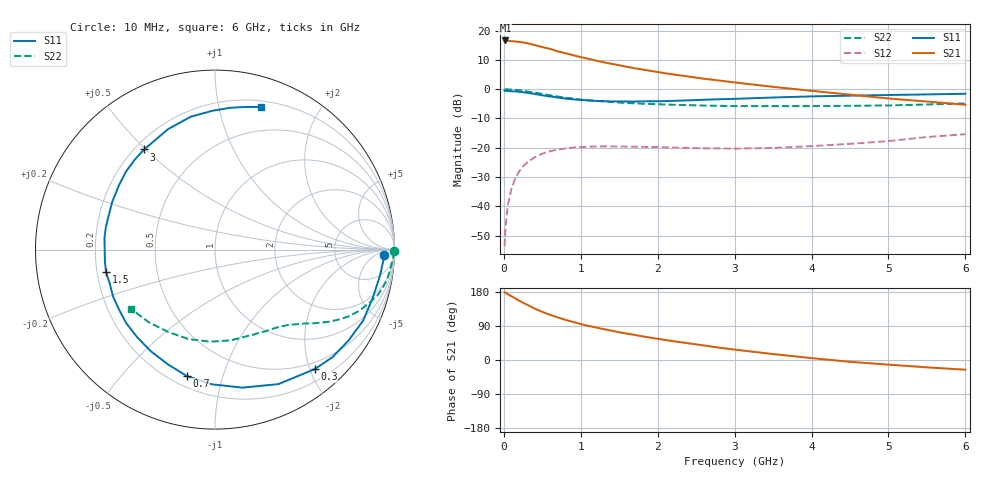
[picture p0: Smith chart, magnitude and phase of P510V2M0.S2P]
! SIEMENS Small Signal Semiconductors
! BFP183
! Si NPN RF Bipolar Junction Transistor in SOT143
! VCE = 10 V  IC = 2 mA
! Common Emitter S-Parameters:  March  1996
# GHz  S  MA  R  50
!  f  S11  S21  S12  S22
! GHz  MAG  ANG  MAG  ANG  MAG  ANG  MAG  ANG
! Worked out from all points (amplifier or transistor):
!   36 points, 10 MHz to 6 GHz, reference 50 ohm
!   highest |S21| = 16.6 dB at 20 MHz (marker M1)
!   |S21| within 3 dB of that: start of sweep to 614.7 MHz
!   unconditionally stable (mu >= 1): 2.182 GHz to 5.881 GHz
!   at 250 MHz: K = 0.11, MSG = 21.2 dB, |S12| = -26.4 dB
!   at 1.4 GHz: K = 0.65, MSG = 14.1 dB, |S12| = -19.5 dB
!   at 6 GHz: K = 0.98, MSG = 5.0 dB, |S12| = -15.4 dB
!   S11 on the Smith chart (normalised r, x): 10 MHz: 26, -12; 300 MHz: 0.39, -2.08; 700 MHz: 0.26, -0.77; 1.5 GHz: 0.24, -0.10; 3 GHz: 0.24, +0.49; 6 GHz: 0.26, +1.34
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0.01  0.9394 -1.7  6.732 178.9  0.0021 81.8  0.9972 -0.6
0.02  0.9401 -3.6  6.767 178.0  0.0041 84.9  0.996 -1.3
0.05  0.9309 -8.8  6.691 174.0  0.0102 87.7  0.9914 -3.2
0.1  0.9193 -17.1  6.589 168.2  0.0204 79.1  0.9826 -6.5
0.2  0.8999 -34.3  6.402 156.5  0.0397 70.2  0.9582 -12.8
0.25  0.8876 -42.4  6.263 151.0  0.048 66.1  0.9399 -15.8
0.3  0.8672 -50.2  6.102 146.2  0.0555 61.8  0.9166 -18.3
0.4  0.8283 -64.8  5.655 135.8  0.0689 54.1  0.8744 -22.9
0.5  0.7843 -78.7  5.211 126.9  0.0796 47.1  0.8291 -26.8
0.6  0.7508 -91.3  4.857 119.3  0.0874 41.3  0.7861 -29.9
0.7  0.7213 -102.7  4.422 112.4  0.0928 36.6  0.7487 -32.5
0.8  0.6902 -112.6  4.1 106.0  0.0973 32.2  0.7165 -34.6
0.9  0.6697 -122.2  3.789 100.5  0.1009 28.5  0.6907 -36.4
1.1  0.6422 -140.5  3.295 89.9  0.1045 23.0  0.6468 -39.5
1.5  0.6203 -168.5  2.554 73.2  0.1051 15.3  0.5896 -45.0
1.8  0.6192 173.7  2.164 62.5  0.1039 12.2  0.5647 -49.1
2.2  0.6316 155.0  1.78 49.7  0.1009 10.3  0.542 -55.1
3  0.6835 125.3  1.302 27.5  0.0968 13.1  0.5137 -69.7
3.5  0.7203 111.3  1.095 15.6  0.0996 16.8  0.5134 -80.1
4.5  0.7735 91.1  0.805 -4.8  0.1167 23.1  0.52 -106.2
5.5  0.8134 77.7  0.615 -19.4  0.1526 24.2  0.5477 -132.3
6  0.8342 72.2  0.542 -25.6  0.1705 21.3  0.5725 -144.8
